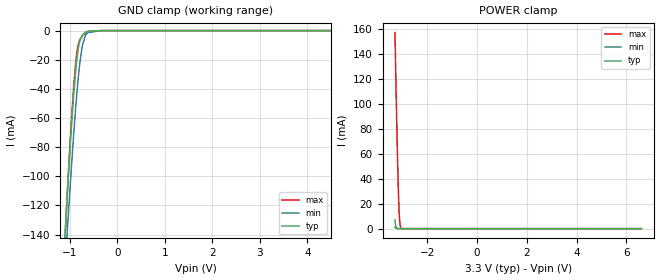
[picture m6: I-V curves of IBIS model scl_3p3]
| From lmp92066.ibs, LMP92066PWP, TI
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|   scl_3p3 Model
[Model]   scl_3p3
Model_type   Input
Vinl = 0.99
Vinh = 2.31
|   typ   min   max
|   (nom PVT)   (fast PVT)   (slow PVT)
C_comp   3.651e-13   3.429e-13   3.983e-13
[Model spec]
|subparameter
Vinl   0.99   0.9   1.08
Vinh   2.31   2.1   2.52
| Where nom  PVT is Nominal Process, 3.3V, 25C
|   Fast PVT is Strong Process,  3.6V, -25C
|   Slow PVT is Weak Process,   3V, 125C
[Voltage Range]   3.3   3   3.6
|Junction Temperature
[Temperature Range]   25   125   -25
[Power Clamp Reference]   3.3   3   3.6
[GND Clamp Reference]   0   0   0
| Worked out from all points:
|   GND clamp passes 1 mA (typ) near -0.65 V on its own axis
|   POWER clamp passes 1 mA (typ) near -3.24 V on its own axis
[GND Clamp]
|   Voltage   I(typ)   I(min)   I(max)
-3.3V     -1.755A    -1.502A    -1.822A
-1.144V   -169.5mA   -187.8mA   -173mA
-1.063V   -119.8mA   -144.4mA   -119.6mA
-1.039V   -106.3mA   -132.2mA   -105mA
-974.4mV  -71.36mA   -99.43mA   -67.36mA
-916.8mV  -44.38mA   -71.84mA   -38.92mA
-866.4mV  -25.04mA   -50mA      -19.97mA
-805.2mV  -9.732mA   -27.78mA   -7.952mA
-735mV    -3.289mA   -10.49mA   -3.505mA
-657.6mV  -1.059mA   -2.715mA   -1.176mA
-326.7mV  -338.4nA   0A         0A
6.6V      0A         0A         0A
[POWER Clamp]
|   Voltage   I(typ)   I(min)   I(max)
-3.3V     7.038mA    1.27mA     157mA
-3.28V    3.622mA    722.8uA    136mA
-3.26V    1.775mA    408.6uA    115.6mA
-3.214V   301uA      105uA      70.39mA
-3.192V   130.6uA    55.89uA    51.66mA
-3.178V   74.62uA    36.69uA    40.3mA
-3.152V   28.05uA    17.49uA    23.36mA
-3.131V   12.11uA    9.219uA    12.69mA
-3.106V   4.536uA    4.305uA    5.172mA
-3.077V   1.48uA     1.731uA    1.541mA
-3.034V   274.6nA    329.3nA    214.7uA
6.6V      0A         0A         0A
